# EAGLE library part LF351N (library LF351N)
IC OPAMP JFET 1 CIRCUIT 8DIP Source: Datasheet
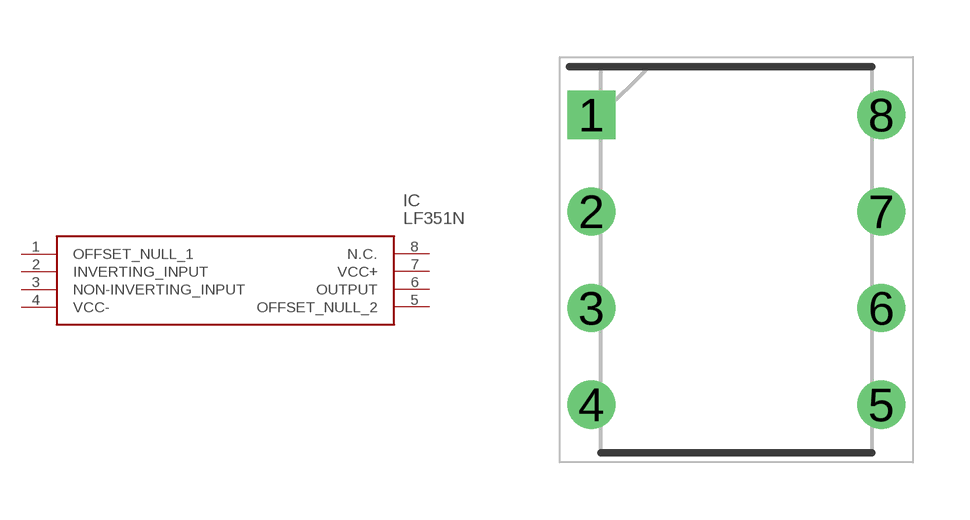
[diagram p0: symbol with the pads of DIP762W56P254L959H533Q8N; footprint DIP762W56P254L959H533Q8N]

Designator prefix IC

## LF351N (Description: IC OPAMP JFET 1 CIRCUIT 8DIP; Height: 5.33mm; Manufacturer_Name: STMicroelectronics; Manufacturer_Part_Number: LF351N; Mouser_Part_Number: 511-LF351N; Mouser_Price-Stock: https://www.mouser.co.uk/ProductDetail/STMicroelectronics/LF351N/?qs=hprEbj%252BdINpkaWu0DIsOeQ%3D%3D)  [DIP762W56P254L959H533Q8N]
1  OFFSET_NULL_1
2  INVERTING_INPUT
3  NON-INVERTING_INPUT
4  VCC-
5  OFFSET_NULL_2
6  OUTPUT
7  VCC+
8  N.C.  nc

## Footprint DIP762W56P254L959H533Q8N (pad centres in mm)
DIP8
drill 0.76 pad 1.16 square: 1 -3.81,3.81
drill 0.76 pad 1.16: 2 -3.81,1.27; 3 -3.81,-1.27; 4 -3.81,-3.81; 5 3.81,-3.81; 6 3.81,-1.27; 7 3.81,1.27; 8 3.81,3.81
